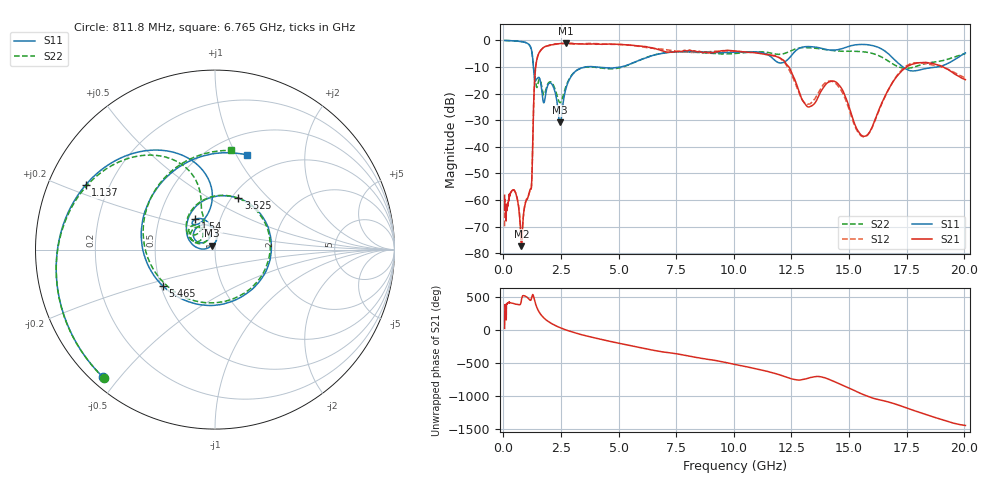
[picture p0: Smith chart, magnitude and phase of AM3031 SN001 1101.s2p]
# Hz S DB R 50
!freq MagS11 AngS11 MagS21 AngS21 MagS12 AngS12 MagS22 AngS22
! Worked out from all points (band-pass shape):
!   1601 points, 50 MHz to 20.05 GHz, reference 50 ohm
!   highest |S21| = -1.05 dB at 2.702 GHz (marker M1); lowest = -77.4 dB at 781.9 MHz (marker M2)
!   |S21| within 3 dB of the highest: 1.587 GHz to 6.928 GHz (5.341 GHz wide, 125 % of centre); 9.4 GHz to 10.13 GHz (729.7 MHz wide, 7.47 % of centre)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
!   lowest |S11| = -30.8 dB at 2.46 GHz (marker M3), VSWR 1.06, Z = 48.2 + j2.2 ohm
!   |S11| at or under -10 dB: 1.298 GHz to 3.552 GHz (2.254 GHz wide, 92.9 % of centre); 4.036 GHz to 5.085 GHz (1.05 GHz wide, 23 % of centre); 17.34 GHz to 18.83 GHz (1.486 GHz wide, 8.22 % of centre)
!   |S22| runs from -23.4 to 0.0 dB; largest |S21 - S12| = 0.067
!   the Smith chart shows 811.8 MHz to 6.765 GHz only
!   S11 on the Smith chart (normalised r, x): 811.8 MHz: 0.03, -0.45; 1.137 GHz: 0.11, +0.23; 1.54 GHz: 0.76, +0.27; 3.525 GHz: 1.07, +0.68; 5.465 GHz: 0.51, -0.24; 6.765 GHz: 0.72, +1.11
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5e7  -0.02 -7.8  -58.25 25.3  -69.90 20.3  -0.04 -7.8
1.35947e8  -0.07 -21.0  -63.97 33.7  -63.35 34.6  -0.06 -21.0
3.696318e8  -0.12 -56.8  -56.49 47.2  -56.36 48.3  -0.12 -57.4
7.819199e8  -0.44 -125.7  -77.39 96.2  -76.58 90.4  -0.42 -125.4
8.117682e8  -0.48 -131.3  -74.16 147.1  -73.07 141.3  -0.47 -130.8
1.005007e9  -0.96 -171.0  -60.04 141.9  -59.68 141.2  -0.94 -169.7
1.137258e9  -1.88 153.4  -56.55 96.9  -56.82 95.0  -1.88 155.4
1.540434e9  -13.92 122.7  -4.74 -82.7  -4.81 -83.2  -14.79 143.3
1.816474e9  -21.11 154.8  -2.28 164.0  -2.34 163.8  -19.32 156.4
2.460443e9  -30.77 127.9  -1.15 36.4  -1.21 36.3  -23.43 135.7
2.702015e9  -18.40 169.5  -1.05 3.5  -1.20 3.6  -17.57 158.9
2.722335e9  -17.78 167.1  -1.06 0.8  -1.20 0.9  -17.07 157.8
3.525348e9  -10.04 65.6  -1.38 -81.4  -1.22 -80.0  -10.11 70.5
5.464583e9  -9.01 -145.4  -1.77 127.9  -1.77 127.7  -9.08 -156.0
6.765401e9  -5.08 71.3  -3.56 38.7  -3.20 42.2  -5.04 80.6
7.401857e9  -4.34 9.9  -4.27 7.7  -3.94 3.4  -4.34 26.6
8.76102e9  -4.42 -108.8  -4.42 -76.0  -4.37 -72.9  -4.73 -93.0
1.056581e10  -4.27 83.4  -4.45 164.0  -4.40 164.9  -4.51 79.9
1.293477e10  -2.64 -102.2  -21.77 -31.3  -21.75 -22.9  -2.74 -95.0
1.559938e10  -1.53 64.6  -35.97 108.0  -36.24 111.4  -4.28 76.9
1.719525e10  -8.99 -58.7  -12.34 -60.1  -11.95 -56.3  -10.09 -90.7
2.005e10  -4.71 71.5  -14.76 -1.9  -14.11 0.2  -4.96 80.5
